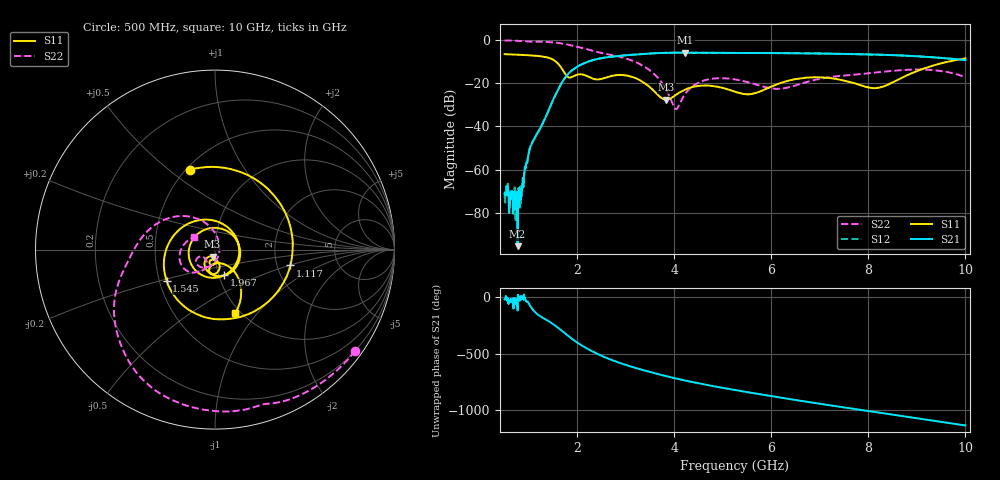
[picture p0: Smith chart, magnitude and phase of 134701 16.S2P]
!  2-Port S-parameters saved by WinCal
! VAR MeasName=S-Parameters (CALIBRATED_DATA) read from VNA (N5242A)
! VAR MeasDate=2013-7-3 16:30:02
! VAR NAME=134701 16
! VAR FILENAME=134701 16.S2P
! VAR DATE=2013-7-3 16:30:02
! VAR PHYS_PORTS=1,2
# Hz S MA R 50
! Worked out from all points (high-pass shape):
!   1601 points, 500 MHz to 10 GHz, reference 50 ohm
!   highest |S21| = -5.95 dB at 4.229 GHz (marker M1); lowest = -95.2 dB at 767.2 MHz (marker M2)
!   |S21| within 3 dB of the highest: 2.396 GHz to 9.812 GHz (7.416 GHz wide, 121 % of centre)
!   lowest |S11| = -27.7 dB at 3.831 GHz (marker M3), VSWR 1.09, Z = 48.5 - j3.79 ohm
!   |S11| at or under -10 dB: 1.552 GHz to 9.667 GHz (8.115 GHz wide, 145 % of centre)
!   |S22| runs from -32.0 to -0.3 dB; largest |S21 - S12| = 0.0028
!   S11 on the Smith chart (normalised r, x): 500 MHz: 0.52, +0.59; 1.117 GHz: 2.37, -0.51; 1.545 GHz: 0.55, -0.21; 1.967 GHz: 1.06, -0.31; 10 GHz: 0.94, -0.78
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5e8  0.4657 107.6  0.0002826 -18.8  0.0002168 -19.8  0.9632 -35.9
7.671875e8  0.4523 62.1  1.73e-05 -116.4  7.661e-05 -13.4  0.9455 -54.9
1.1175e9  0.4291 -11.8  0.005272 -125.8  0.005255 -127.0  0.9064 -78.3
1.360938e9  0.3938 -78.6  0.01776 159.9  0.01778 159.9  0.8906 -96.2
1.545e9  0.3207 -147.2  0.05278 108.8  0.05264 108.6  0.8593 -110.5
1.729062e9  0.1765 108.8  0.1249 47.1  0.1247 46.9  0.8014 -124.9
1.966562e9  0.1527 -70.2  0.2274 -31.5  0.227 -31.6  0.7041 -141.6
2.085312e9  0.1595 -128.6  0.2703 -64.6  0.2697 -64.7  0.6543 -149.4
2.37625e9  0.1219 100.1  0.3529 -132.9  0.352 -132.9  0.5337 -165.6
2.702812e9  0.1458 -18.7  0.4065 166.1  0.4061 166.1  0.4438 178.4
3.18375e9  0.1323 -105.0  0.4554 97.2  0.4556 97.2  0.3122 145.9
3.670625e9  0.05222 -130.6  0.4935 39.6  0.493 39.6  0.1286 101.9
3.830938e9  0.04125 -109.2  0.4998 22.4  0.4999 22.4  0.07093 80.1
4.032812e9  0.05361 -87.7  0.5036 1.9  0.5034 1.8  0.02515 -3.0
4.22875e9  0.07125 -87.4  0.5043 -16.8  0.5041 -16.9  0.05752 -81.6
4.6325e9  0.08813 -103.1  0.5003 -52.2  0.5003 -52.3  0.1172 -120.7
5.25e9  0.06324 -112.2  0.4955 -100.5  0.4956 -100.6  0.1215 -150.1
6.08125e9  0.09054 -73.8  0.4941 -159.9  0.4939 -159.9  0.07364 -140.1
6.835312e9  0.1358 -92.4  0.4854 148.9  0.4854 148.9  0.114 -117.2
7.625e9  0.1056 -106.7  0.469 97.6  0.4691 97.6  0.1535 -127.0
8.420625e9  0.09395 -58.7  0.4451 46.1  0.4439 46.2  0.1882 -138.6
1e10  0.3716 -72.3  0.342 -53.8  0.3437 -53.7  0.1364 149.2
